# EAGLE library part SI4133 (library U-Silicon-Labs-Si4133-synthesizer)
RF Synthesizer w/ integrated VCOs (RF1/RF2/IF OUT)
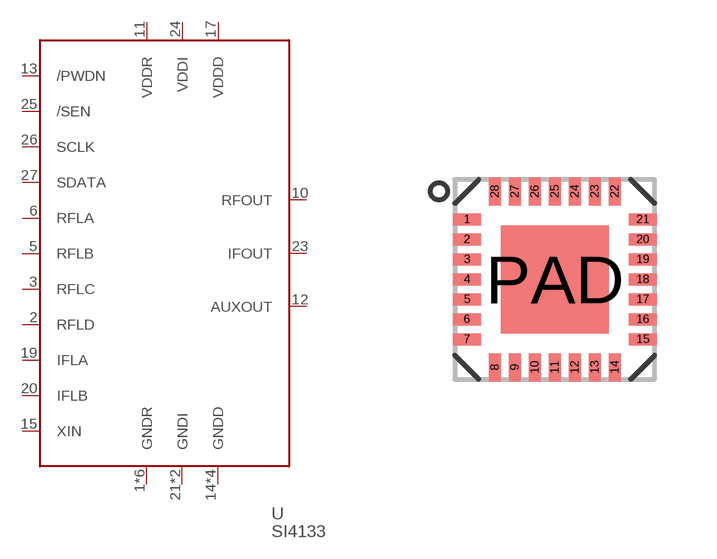
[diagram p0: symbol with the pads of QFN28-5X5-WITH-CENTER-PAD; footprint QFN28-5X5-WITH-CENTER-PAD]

Designator prefix U

## SI4133  [QFN28-5X5-WITH-CENTER-PAD]
1  GNDR  pwr
2  RFLD  in
3  RFLC  in
4  GNDR  pwr
5  RFLB  in
6  RFLA  in
7  GNDR  pwr
8  GNDR  pwr
9  GNDR  pwr
10  RFOUT  out
11  VDDR  pwr
12  AUXOUT  out
13  /PWDN  in
14  GNDD  pwr
15  XIN  in
16  GNDD  pwr
17  VDDD  pwr
18  GNDD  pwr
19  IFLA  in
20  IFLB  in
21  GNDI  pwr
22  GNDI  pwr
23  IFOUT  out
24  VDDI  pwr
25  /SEN  in
26  SCLK  in
27  SDATA  in
28  GNDR  pwr
PAD  GNDD  pwr

## Footprint QFN28-5X5-WITH-CENTER-PAD (pad centres in mm)
smd 0.7 x 0.3: 1 -2.2,1.5; 2 -2.2,1; 3 -2.2,0.5; 4 -2.2,0; 5 -2.2,-0.5; 6 -2.2,-1; 7 -2.2,-1.5; 15 2.2,-1.5; 16 2.2,-1; 17 2.2,-0.5; 18 2.2,0; 19 2.2,0.5; 20 2.2,1; 21 2.2,1.5
smd 0.3 x 0.7: 8 -1.5,-2.2; 9 -1,-2.2; 10 -0.5,-2.2; 11 0,-2.2; 12 0.5,-2.2; 13 1,-2.2; 14 1.5,-2.2; 22 1.5,2.2; 23 1,2.2; 24 0.5,2.2; 25 0,2.2; 26 -0.5,2.2; 27 -1,2.2; 28 -1.5,2.2
smd 2.7 x 2.7: PAD 0,0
